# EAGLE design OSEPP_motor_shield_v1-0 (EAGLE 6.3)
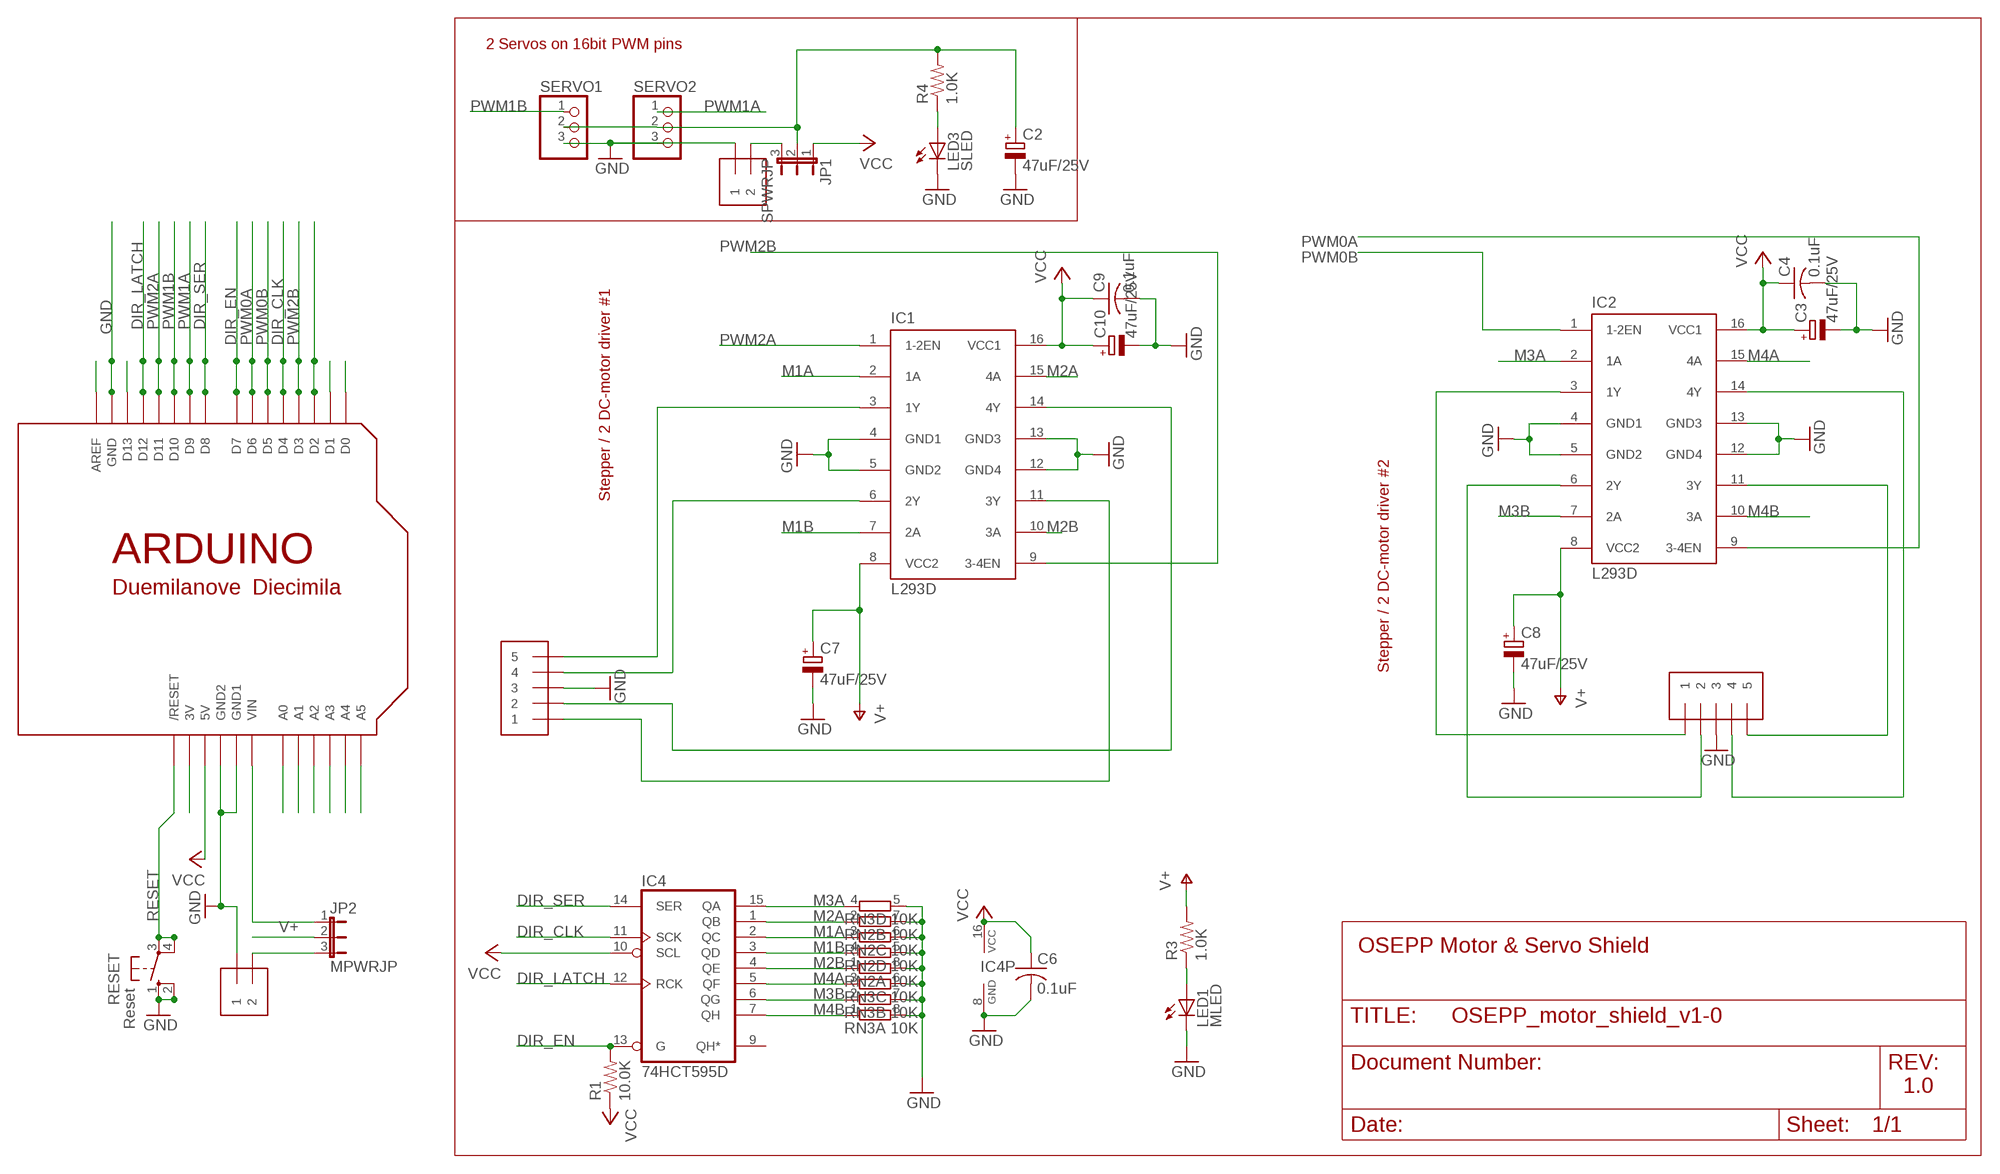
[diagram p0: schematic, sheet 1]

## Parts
C2  47uF/25V  CPOL-EUD  [PANASONIC_D]
C3  47uF/25V  CPOL-EUD  [PANASONIC_D]
C4  0.1uF  C-USC0603  [C0603]
C6  0.1uF  C-USC0603  [C0603]
C7  47uF/25V  CPOL-EUD  [PANASONIC_D]
C8  47uF/25V  CPOL-EUD  [PANASONIC_D]
C9  0.1uF  C-USC0603  [C0603]
C10  47uF/25V  CPOL-EUD  [PANASONIC_D]
IC1  L293D  L293E  [DIL16]
IC2  L293D  L293E  [DIL16]
IC4  74HCT595D  [SO16]
J1  1X5  [1X05-3.5MM]
J2  1X5  [1X05-3.5MM]
J3  1X2-3.5MM  [1X2-3.5MM]
J5  1X2-3.5MM  [1X2-3.5MM]
JP1  SPWRJP  JP2E  [JP2]
JP2  MPWRJP  JP2E  [JP2]
LED1  MLED  LEDCHIPLED_0805  [CHIPLED_0805]
LED3  SLED  LEDCHIPLED_0805  [CHIPLED_0805]
R1  10.0K  R-US_R0603  [R0603]
R3  1.0K  R-US_R0603  [R0603]
R4  1.0K  R-US_R0603  [R0603]
RESET  Reset  10-XX  [B3F-10XX]
RN2  10K  4R-NCAY16  [CAY16]
RN3  10K  4R-NCAY16  [CAY16]
SERVO1  PINHD-1X3  [1X03]
SERVO2  PINHD-1X3  [1X03]
U$1  ARDUINO-NOHOLE  [ARDUINO-NOHOLE]

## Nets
9V: JP2.1 U$1.VIN
DIR_CLK: IC4.11(SCK) U$1.D4
DIR_EN: IC4.13(G) R1.2 U$1.D7
DIR_LATCH: IC4.12(RCK) U$1.D12
DIR_SER: IC4.14(SER) U$1.D8
GND [power]: C2.- C3.- C4.2 C6.2 C7.- C8.- C9.2 C10.- IC1.4(GND1) IC1.5(GND2) IC1.12(GND4) IC1.13(GND3) IC2.4(GND1) IC2.5(GND2) IC2.12(GND4) IC2.13(GND3) IC4.8(GND) J1.3 J2.3 J3.1 J5.1 LED1.C LED3.C RESET.1(S) RESET.2(S1) RN2.5 RN2.6 RN2.7 RN2.8 RN3.5 RN3.6 RN3.7 RN3.8 SERVO1.3 SERVO2.3 U$1.GND U$1.GND1 U$1.GND2
M1A: IC1.2(1A) IC4.2(QC) RN2.3
M1B: IC1.7(2A) IC4.3(QD) RN2.4
M2A: IC1.15(4A) IC4.1(QB) RN2.2
M2B: IC1.10(3A) IC4.4(QE) RN2.1
M3A: IC2.2(1A) IC4.15(QA) RN3.4
M3B: IC2.7(2A) IC4.6(QG) RN3.2
M4A: IC2.15(4A) IC4.5(QF) RN3.3
M4B: IC2.10(3A) IC4.7(QH) RN3.1
N$1: IC1.3(1Y) J1.5
N$2: U$1.A0
N$3: U$1.A1
N$4: U$1.A2
N$5: U$1.A3
N$6: U$1.A4
N$7: IC2.3(1Y) J2.1
N$8: IC2.6(2Y) J2.2
N$9: IC2.11(3Y) J2.5
N$10: U$1.D2
N$11: U$1.D1
N$12: U$1.D0
N$13: U$1.A5
N$14: U$1.AREF
N$15: U$1.D13
N$16: LED1.A R3.1
N$17: U$1.3V
N$18: C2.+ JP1.2 R4.2 SERVO1.2 SERVO2.2
N$19: J3.2 JP2.3
N$20: IC2.14(4Y) J2.4
N$21: LED3.A R4.1
N$22: J5.2 JP1.3
N$31: IC1.6(2Y) J1.4
N$32: IC1.11(3Y) J1.1
N$33: IC1.14(4Y) J1.2
PWM0A: IC2.9(3-4EN) U$1.D6
PWM0B: IC2.1(1-2EN) U$1.D5
PWM1A: SERVO2.1 U$1.D9
PWM1B: SERVO1.1 U$1.D10
PWM2A: IC1.1(1-2EN) U$1.D11
PWM2B: IC1.9(3-4EN) U$1.D3
RESET: RESET.3(P) RESET.4(P1) U$1.RESET(/RESET)
V+: C7.+ C8.+ IC1.8(VCC2) IC2.8(VCC2) JP2.2 R3.2
VCC: C3.+ C4.1 C6.1 C9.1 C10.+ IC1.16(VCC1) IC2.16(VCC1) IC4.10(SCL) IC4.16(VCC) JP1.1 R1.1 U$1.5V
Unconnected: IC4.9(QH*)

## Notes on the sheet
- 2 Servos on 16bit PWM pins
- Stepper / 2 DC-motor driver #1
- Stepper / 2 DC-motor driver #2
- OSEPP Motor & Servo Shield
- 1.0

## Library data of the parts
C2 C3 C7 C8 C10 = rcl:CPOL-EU: POLARIZED CAPACITOR, European symbol
C4 C6 C9 = rcl:C-US: CAPACITOR, American symbol
IC1 IC2 = texas:L293E: TI DEVICE; MF: Arrow Electronics; MPN: L293E; OC_FARNELL: 1467711; OC_NEWARK: 89K0732
IC4 = 74xx-eu:74*595: 8-bit SHIFT REGISTER, output latch
J1 J2 = adafruit:1X5
J3 J5 = adafruit:1X2: 3.5mm Terminal block
JP1 JP2 = jumper:JP2E: JUMPER
LED1 LED3 = led:LED: LED
R1 R3 R4 = resistor:R-US_: RESISTOR, American symbol
RESET = switch-omron:10-XX: OMRON SWITCH; MPN: B3F-1000; OC_FARNELL: 176432; OC_NEWARK: 36M3542
RN2 RN3 = resistor-dil:4R-N: Array Chip Resistor Source: RS Component / Phycomp; OC_FARNELL: unknown; OC_NEWARK: unknown
SERVO1 SERVO2 = pinhead:PINHD-1X3: PIN HEADER
U$1 = adafruit:ARDUINO: Arduino Diecimila/Duemilanove Make a shield with ease, this package has all the named pins as well as the two mounting drill holes and an outline of the USB and DC power connector. The outline is on the DIMENSION layer, so if your board house uses it they will cut the outline to match.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

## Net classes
1 power: width 0.61 mm

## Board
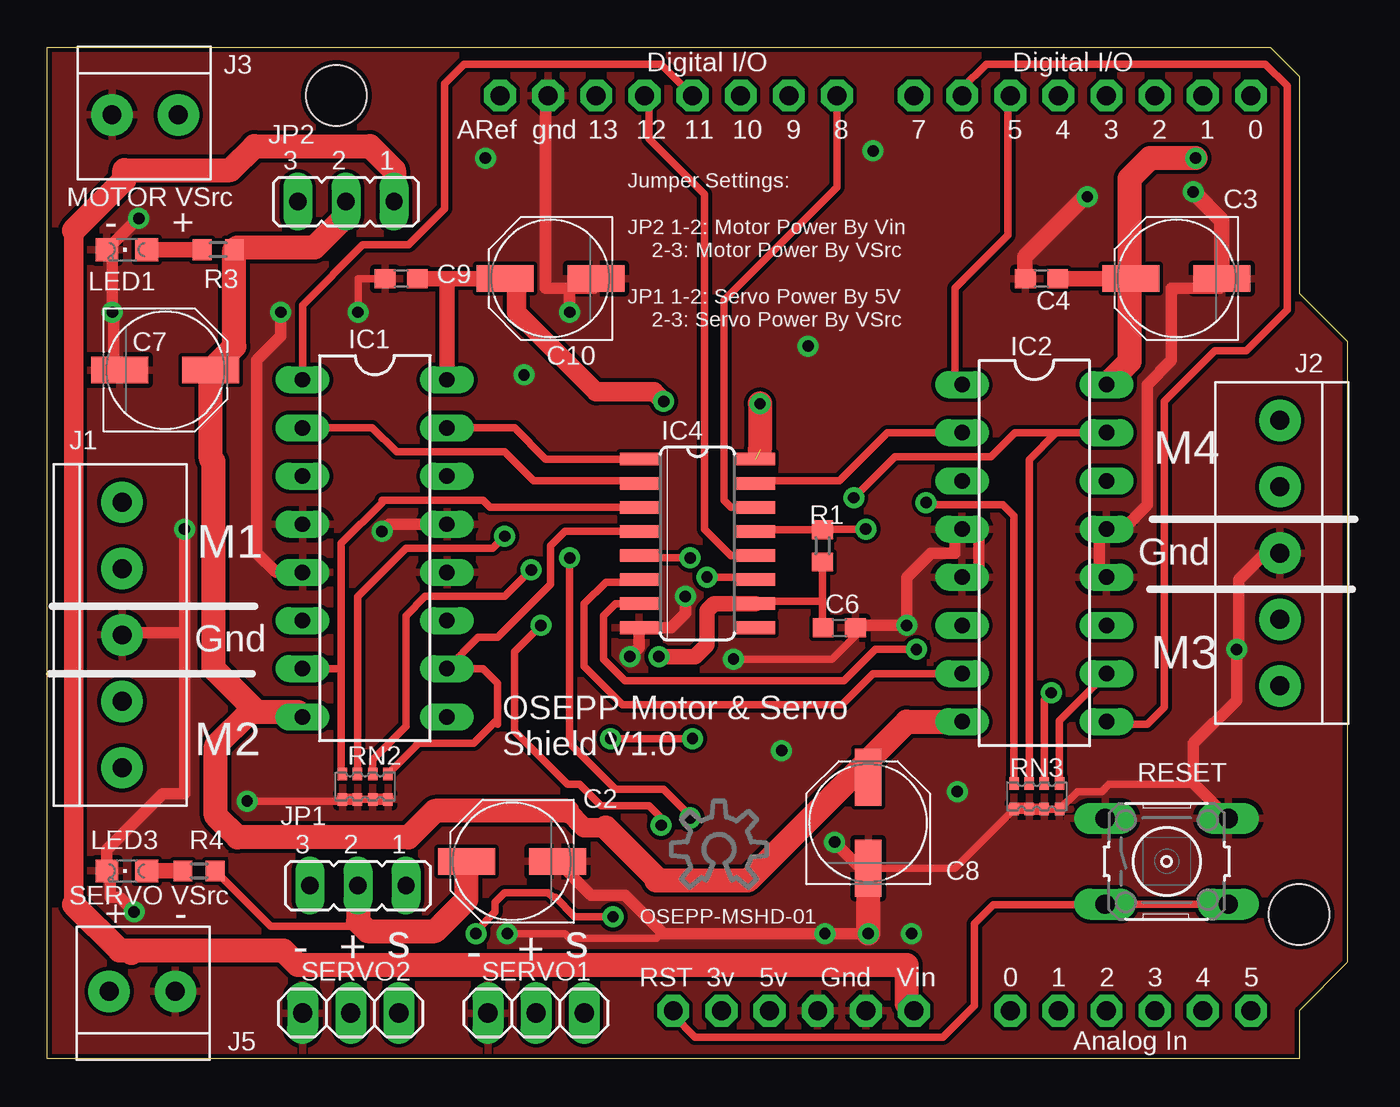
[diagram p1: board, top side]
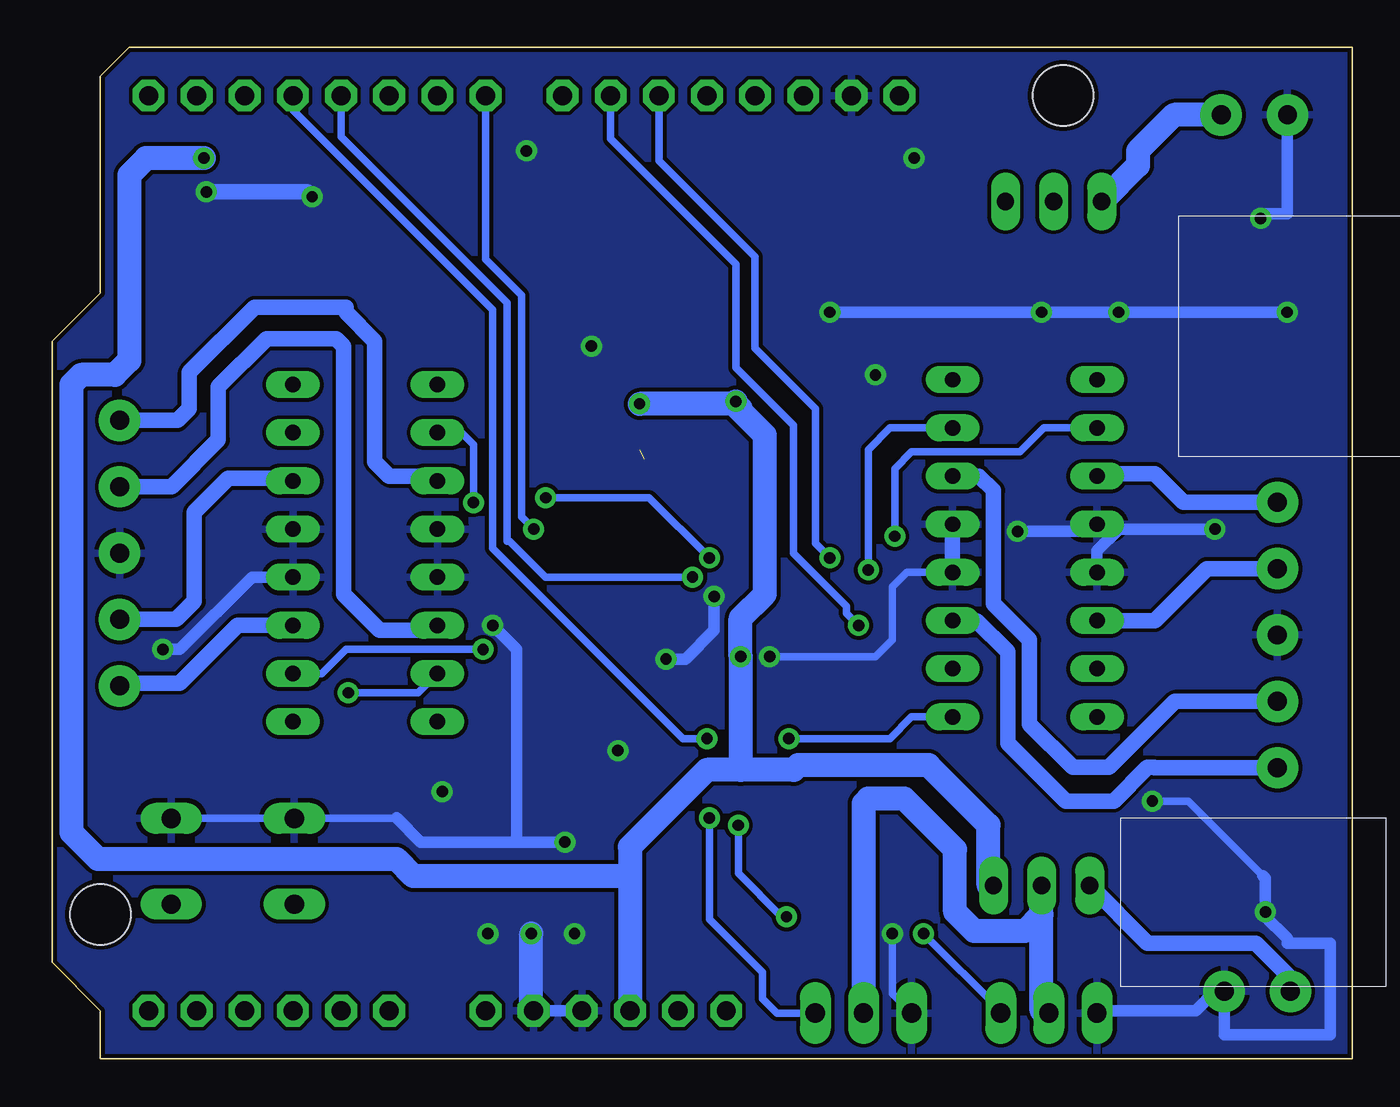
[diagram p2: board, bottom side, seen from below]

Size 68.58 x 53.34 mm. Coordinates in mm from the lower left corner, seen from the top.
Outline: 0,0 0,53.34 64.52,53.34 66.04,51.82 66.04,40.39 68.58,37.85 68.58,5.08 66.04,2.54 66.04,0 0,0
Copper layers (1*16): Top 0.035mm / dielectric 1.5mm / Bottom 0.035mm
Design rules "SparkFun": minimum track width 8mil, minimum drill 20mil, track to track 8mil, track to pad 8mil, pad to pad 8mil, via to via 8mil, smd to smd 8mil, copper to edge 10mil, drill to drill 8mil, minimum pad ring 12mil, minimum via ring 10mil, stop-mask expansion 4mil, vias tented up to drill 25mil, thermal gap 10mil
Holes 3.2 mm at 66.04,7.62 15.24,50.8

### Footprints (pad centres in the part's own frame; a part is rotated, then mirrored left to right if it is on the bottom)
PANASONIC_D = smd 3 x 1.4: + 2.4,0; - -2.4,0
C0603 = smd 1.1 x 1: 1 -0.85,0; 2 0.85,0
DIL16 = drill 0.813 long: 1 -8.89,-3.81; 2 -6.35,-3.81; 3 -3.81,-3.81; 4 -1.27,-3.81; 5 1.27,-3.81; 6 3.81,-3.81; 7 6.35,-3.81; 8 8.89,-3.81; 9 8.89,3.81; 10 6.35,3.81; 11 3.81,3.81; 12 1.27,3.81; 13 -1.27,3.81; 14 -3.81,3.81; 15 -6.35,3.81; 16 -8.89,3.81
SO16 = smd 0.66 x 2.032: 1 -4.445,-3.073; 2 -3.175,-3.073; 3 -1.905,-3.073; 4 -0.635,-3.073; 5 0.635,-3.073; 6 1.905,-3.073; 7 3.175,-3.073; 8 4.445,-3.073; 9 4.445,3.073; 10 3.175,3.073; 11 1.905,3.073; 12 0.635,3.073; 13 -0.635,3.073; 14 -1.905,3.073; 15 -3.175,3.073; 16 -4.445,3.073
1X05-3.5MM = drill 1 pad 2.184: 1 7,0; 2 3.5,0; 3 0,0; 4 -3.5,0; 5 -7,0
1X2-3.5MM = drill 1 pad 2.184: 1 1.8,0; 2 -1.7,0
JP2 = drill 0.914 long: 1 -2.54,0; 2 0,0; 3 2.54,0
CHIPLED_0805 = smd 1.2 x 1.2: A 0,-1.05; C 0,1.05
R0603 = smd 1 x 1.1: 1 -0.85,0; 2 0.85,0
B3F-10XX = drill 1.016 long: 1 -3.251,2.261; 2 3.251,2.261; 3 -3.251,-2.261; 4 3.251,-2.261
CAY16 = smd 0.5 x 0.65: 1 -1.2,-0.675; 2 -0.4,-0.675; 3 0.4,-0.675; 4 1.2,-0.675; 5 1.2,0.675; 6 0.4,0.675; 7 -0.4,0.675; 8 -1.2,0.675
1X03 = drill 1.016 long: 1 -2.54,0; 2 0,0; 3 2.54,0
ARDUINO-NOHOLE = drill 1 pad 1.676 octagon: 3V 35.56,2.54; 5V 38.1,2.54; A0 50.8,2.54; A1 53.34,2.54; A2 55.88,2.54; A3 58.42,2.54; A4 60.96,2.54; A5 63.5,2.54; AREF 23.876,50.8; D0 63.5,50.8; D1 60.96,50.8; D2 58.42,50.8; D3 55.88,50.8; D4 53.34,50.8; D5 50.8,50.8; D6 48.26,50.8; D7 45.72,50.8; D8 41.656,50.8; D9 39.116,50.8; D10 36.576,50.8; D11 34.036,50.8; D12 31.496,50.8; D13 28.956,50.8; GND 26.416,50.8; GND1 43.18,2.54; GND2 40.64,2.54; RESET 33.02,2.54; VIN 45.72,2.54

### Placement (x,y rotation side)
C2  24.51,10.41 180 top
C3  59.56,41.15 180 top
C4  52.45,41.15 180 top
C6  41.78,22.73 0 top
C7  6.22,36.32 0 top
C8  43.31,12.45 90 top
C9  18.67,41.15 180 top
C10  26.54,41.15 180 top
E$1  [OSHWLOGO_TOL_0.2]  35.43,11.05 0 top
IC1  17.27,26.92 270 top
IC2  52.07,26.67 270 top
IC4  34.29,27.18 270 top
J1  3.94,22.35 270 top
J2  65.02,26.67 90 top
J3  5.21,49.78 180 top
J5  4.95,3.56 0 top
JP1  16.38,9.14 180 top
JP2  15.75,45.21 180 top
LED1  4.19,42.67 90 top
LED3  4.19,9.91 90 top
R1  40.89,27.05 90 top
R3  9.02,42.67 0 top
R4  8,9.91 0 top
RESET  59.05,10.41 0 top
RN2  16.76,14.35 180 top
RN3  52.2,13.84 180 top
SERVO1  25.78,2.41 180 top
SERVO2  16,2.41 180 top
U$1  0,0 0 top

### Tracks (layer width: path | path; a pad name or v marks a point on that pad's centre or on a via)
9V
  Top 1.016: 1.4,8.13 1.4,43.69
  Top 1.27: U$1.VIN 45.34,2.92 45.34,4.95 13.21,4.95 12.45,5.71 4.57,5.71 | 1.4,43.69 4.06,46.35 4.06,46.86 9.65,46.86 10.92,48.13 17.02,48.13 18.29,46.86 JP2.1 | 4.44,5.59 4.57,5.71 | 1.4,8.13 3.81,5.71 4.57,5.71
DIR_CLK  (via drill 0.6)
  Top 0.406: v34.8,25.4 37.24,25.4 IC4.11
  Bottom 0.406: v34.8,25.4 42.55,25.4 44.45,27.3 44.58,27.3 44.58,39.88 53.34,48.64 U$1.D4
DIR_EN  (via drill 0.6)
  Top 0.406: IC4.13 37.45,27.9 R1.2 40.93,27.94 v43.18,27.94
  Bottom 0.406: U$1.D7 45.72,42.16 43.81,40.26 43.81,28.57 v43.18,27.94
DIR_LATCH
  Top 0.406: IC4.12 36.07,26.54 34.67,27.94 34.67,45.59 31.75,48.51 31.75,50.55 U$1.D12
DIR_SER
  Top 0.406: IC4.14 36.07,29.08 35.69,29.46 35.69,40.01 41.66,45.97 U$1.D8
GND  (via drill 0.6)
  Top 0.406: C9.2 16.38,41.15 v16.38,39.37 | RN3.7 RN3.8 54.33,14.1 55.63,14.1 56.01,14.48 60.58,14.48 | RN3.6 RN3.5 47.88,10.05 C8.- | RN2.7 RN2.6 | RN2.5 15.48,13.59 v10.54,13.59 | 32.38,6.6 32.13,6.35 27.56,6.35 27.3,6.6 v24.26,6.6 | v36.2,21.08 41.4,21.08 42.63,22.31 C6.2
  Top 0.61: 27.56,40.64 26.29,40.64 26.29,50.8 U$1.GND | 27.56,40.64 28.83,40.64 | 3.43,36.83 3.5,36.73 | 3.5,36.73 C7.- | IC2.12 55.5,25.4 55.5,27.94 IC2.13 56.77,27.94 58.04,29.21 58.04,35.56 59.31,36.83 59.31,40.64 61.85,40.64 C3.- | C6.2 42.8,22.86 v45.34,22.86 45.34,25.4 46.61,26.67 47.88,26.67 47.88,27.94 IC2.4 49.15,27.94 49.15,25.4 IC2.5 | C8.- 42.8,10.16 v41.53,11.43 | C2.- 28.69,8.64 30.48,8.64 32.38,6.73 32.38,6.6 v41.02,6.6 v43.31,6.6 | RN2.6 RN2.5 | RN2.7 RN2.8 | RN3.7 RN3.6 51.76,13.21 50.93,13.21 | IC1.5 12.06,25.65 11.05,26.67 11.05,36.83 12.32,38.1 v12.32,39.37 | v17.65,27.81 18.03,28.19 IC1.13 | J2.3 64.26,26.67 62.87,25.27 62.87,21.72 v62.74,21.59 62.74,18.92 60.45,16.64 60.45,14.53 RESET.2 | 3.5,36.73 3.5,39.3 v3.43,39.37 3.43,42.16 3.14,42.45 LED1.C 4.79,44.32 v4.83,44.32 | v7.24,27.94 7.24,22.48 | 7.24,22.48 7.24,13.97 6.1,13.97 3.14,11.02 LED3.C 3.3,9.74 3.3,8.51 3.81,8.51 v4.57,7.75 | J1.3 4.06,22.48 7.24,22.48 | v30.73,21.21 31.22,21.69 IC4.8 32.89,22.73 33.66,23.5 v33.66,24.38 | C10.- 29.72,41.15 | v27.56,39.37 27.56,40.64
  Top 0.813: C4.2 51.56,41.19 51.56,42.29 54.74,45.47 v54.86,45.47 | v60.45,45.72 61.96,44.21 C3.-
  Top 1.27: v43.31,6.6 C8.-
  Bottom 0.406: IC1.12 23.5,25.65 24.26,24.89 24.26,22.1 25.15,21.21 v30.73,21.21 | v10.54,13.59 8.64,13.59 4.7,9.65 | 50.42,12.7 50.44,12.68 RESET.1 RESET.2 | 61.85,12.7 61.98,12.7 | SERVO1.3 24.26,3.43 v24.26,6.6
  Bottom 0.61: SERVO2.3 13.59,2.54 8.25,2.54 7.24,3.56 J5.1 6.73,3.56 6.73,1.27 1.14,1.27 1.14,6.1 3.43,6.1 3.43,6.35 4.57,7.49 v4.57,7.75 4.57,9.53 4.7,9.65 | v7.24,27.94 12.32,27.94 | U$1.GND1 U$1.GND2 40.26,2.54 | 44.07,11.43 49.15,11.43 50.42,12.7 | 44.07,11.43 44.07,21.59 v45.34,22.86 | IC2.12 58.04,25.4 61.85,21.59 v62.74,21.59 | v36.2,21.08 35.18,21.08 33.66,22.61 v33.66,24.38 | 12.32,27.94 12.57,28.19 IC1.4 13.84,27.81 v17.65,27.81 | 12.32,27.94 13.46,26.8 IC1.5 | v3.43,39.37 v12.32,39.37 v16.38,39.37 v27.56,39.37 | v41.53,11.43 44.07,11.43 | v4.83,44.32 4.57,44.58 3.43,44.58 3.41,44.6 J3.1
  Bottom 0.813: v54.86,45.47 55.12,45.72 v60.45,45.72 | IC1.13 IC1.12
  Bottom 1.27: U$1.GND1 43.31,2.67 v43.31,6.6
  other vias: 23.11,47.5 43.56,47.88 48.01,14.1 38.73,16.26 40.13,37.59 25.15,36.07 45.59,6.6
  pour Bottom: -0.64,53.85 -0.64,-1.02 69.22,-1.02 69.22,53.98 -0.64,53.98
  pour Top: -0.64,53.98 -0.76,53.85 -0.64,-1.02 69.22,-1.02 69.22,53.98
M1A  (via drill 0.6)
  Top 0.254: 31.09,30.48 IC4.2
  Top 0.406: IC1.2 17.14,33.27 18.41,32 24.13,32 25.65,30.48 31.09,30.48 | RN2.3 16.36,24.36 18.92,26.92 23.5,26.92 v24.13,27.56
  Bottom 0.406: v24.13,27.56 24.13,31.11 23.24,32 17.53,32 16.26,33.27 IC1.2
M1B
  Top 0.406: IC1.7 15.49,20.57 | 15.49,20.57 15.49,27.18 17.65,29.34 17.65,29.46 22.99,29.46 23.37,29.08 IC4.3 | RN2.4 15.49,15.1 15.49,20.57
M2A  (via drill 0.6)
  Top 0.406: IC1.15 24.64,33.27 26.29,31.62 IC4.1 | RN2.2 17.16,15.77 18.92,17.53 18.92,23.37 19.94,24.38 24.13,24.38 v25.53,25.78
  Bottom 0.406: v25.53,25.78 25.53,32.13 24.38,33.27 IC1.15
M2B
  Top 0.406: IC4.4 27.3,27.81 26.54,27.05 26.54,25.02 23.75,22.23 22.73,22.23 IC1.10 22.99,20.57 23.75,19.81 23.75,18.16 23.75,17.91 | 23.75,17.65 23.75,17.91 | RN2.1 19.47,16.53 19.47,16.55 19.56,16.64 22.48,16.64 23.75,17.91
M3A  (via drill 0.6)
  Top 0.254: 37.49,30.48 IC4.15
  Top 0.406: IC2.2 44.32,33.02 41.78,30.48 37.49,30.48 | RN3.4 51,28.63 50.42,29.21 46.48,29.21 v46.35,29.34
  Bottom 0.406: 47.24,33.02 IC2.2 46.99,33.02 46.35,32.38 v46.35,29.34
M3B  (via drill 0.6)
  Top 0.254: IC2.7 48.39,20.32
  Top 0.406: IC2.7 43.56,20.32 41.91,18.67 30.35,18.67 28.32,20.7 28.32,24 29.46,25.15 31.09,25.15 IC4.6 | RN3.2 52.6,18.94 v52.96,19.3
  Bottom 0.406: v52.96,19.3 49.28,19.3 IC2.7
M4A  (via drill 0.6)
  Top 0.406: IC2.15 53.21,33.02 | 53.21,33.02 51.05,33.02 49.78,31.75 44.7,31.75 v42.55,29.59 | v33.91,26.42 31.34,26.42 IC4.5 | RN3.3 51.8,31.6 53.21,33.02
  Bottom 0.406: v42.55,29.59 37.08,29.59 v33.91,26.42
M4B  (via drill 0.6)
  Top 0.406: RN3.1 53.4,17.84 IC2.10 | IC4.7 29.97,24 29.34,23.37 29.34,21.08 30.48,19.94 42.04,19.94 43.69,21.59 v45.85,21.59
  Bottom 0.406: v45.85,21.59 53.09,21.59 54.36,20.32 IC2.10 55.63,20.07
N$1
  Bottom 0.813: J1.5 8.9,29.35 10.41,30.86 13.33,30.86 IC1.3
N$7
  Bottom 0.813: J2.1 61.96,33.67 61.34,34.29 61.34,36.2 57.91,39.62 53.09,39.62 53.09,39.37 51.56,37.85 51.56,31.5 50.8,30.73 48.51,30.73 IC2.3
N$8
  Bottom 0.813: J2.2 62.29,30.17 59.82,32.64 59.82,35.43 57.28,37.97 53.59,37.97 53.21,37.59 53.21,24.51 51.31,22.61 48.51,22.61 IC2.6
N$9
  Bottom 0.813: IC2.11 58.8,22.86 61.85,19.81 64.88,19.81 J2.5
N$16
  Top 0.813: LED1.A R3.1
N$18
  Top 0.406: R4.2 11.77,6.99 16.38,6.99 JP1.2
  Top 1.27: JP1.2 16.38,7.24 16.89,6.73 20.45,6.73 22.11,8.39 C2.+
  Bottom 1.27: SERVO2.2 16.13,2.29 16.38,2.54 JP1.2 16.38,7.62 17.27,6.73 19.94,6.73 20.95,7.75 20.95,11.05 23.62,13.72 25.53,13.72 25.78,13.46 SERVO1.2
N$19
  Bottom 1.27: J3.2 9.4,49.78 11.3,47.88 11.3,47.12 JP2.3
N$20
  Bottom 0.813: J2.4 62.05,23.17 61.09,24.13 61.09,28.83 59.31,30.61 56.01,30.61 IC2.14
N$21
  Top 0.813: R4.1 LED3.A
N$22
  Bottom 0.813: J5.2 3.25,4.27 5.08,6.1 10.79,6.1 JP1.3
N$31
  Bottom 0.813: J1.4 7.68,25.85 10.41,23.11 IC1.6
N$32
  Bottom 0.813: J1.1 10.43,15.35 10.44,15.37 10.79,15.37 12.57,13.59 15.11,13.59 18.16,16.64 18.16,21.46 19.81,23.11 IC1.11
N$33
  Bottom 0.813: J1.2 9.34,18.85 12.83,15.37 14.73,15.37 17.02,17.65 17.02,22.1 18.92,24 18.92,29.97 19.68,30.73 IC1.14 20.83,30.48
PWM0A
  Top 0.406: U$1.D6 48.26,51.18 49.53,52.45 64.26,52.45 65.41,51.31 65.41,39.5 63.25,37.34 61.59,37.34 58.93,34.67 58.93,18.54 58.04,17.65 56.01,17.65 IC2.9
PWM0B
  Top 0.406: U$1.D5 50.67,50.93 50.67,43.43 47.88,40.64 47.88,35.94 IC2.1
PWM1A  (via drill 0.6)
  Top 0.406: v22.61,6.6 22.61,6.73 23.62,7.75 23.62,8.26 24.13,8.76 26.42,8.76 26.67,8.51 26.8,8.51 27.81,7.49 v29.84,7.49 | v32.38,12.32 32.38,12.7 31.75,13.34 29.21,13.34 28.07,14.48 27.43,14.48 24.64,17.27 24.64,21.46 v26.04,22.86
  Bottom 0.406: U$1.D9 39.12,48.51 32.51,41.91 32.51,36.45 29.46,33.4 29.46,26.67 26.67,23.88 26.67,23.5 v26.04,22.86 | v22.61,6.6 18.54,2.54 SERVO2.1 | 29.97,7.62 v29.84,7.49 30.1,7.49 32.38,9.78 v32.38,12.32
PWM1B  (via drill 0.6)
  Top 0.406: v27.56,26.42 27.56,16.64 29.97,14.22 32.51,14.22 33.91,12.83 v33.91,12.7
  Bottom 0.406: SERVO1.1 30.35,2.41 31.11,3.17 31.11,4.57 33.91,7.37 v33.91,12.7 | v27.56,26.42 28.32,27.18 28.32,34.29 31.5,37.47 31.5,42.29 36.58,47.37 U$1.D10
PWM2A
  Top 0.406: IC1.1 13.46,39.75 16.64,42.93 19.05,42.93 20.95,44.83 20.95,51.44 21.97,52.45 32.38,52.45 U$1.D11
PWM2B  (via drill 0.6)
  Top 0.406: v29.72,16.89 v34.04,16.89
  Bottom 0.406: v29.72,16.89 24.38,16.89 23.24,18.03 IC1.9 | v34.04,16.89 35.31,16.89 45.34,26.92 45.34,39.5 55.88,50.04 U$1.D3
RESET
  Top 0.406: U$1.RESET 33.02,2.29 34.16,1.14 47.24,1.14 48.9,2.79 48.9,7.11 49.91,8.13 55.78,8.13 RESET.3 RESET.4
V+
  Top 0.813: 9.91,40.26 9.91,42.63 | 9.91,42.63 R3.2 | 9.91,42.63 9.91,42.67 10.03,42.8 | 15.75,44.45 JP2.2 | C8.+ 43.31,15.75 | 48.01,17.53 IC2.8
  Top 1.016: 27.43,13.08 28.32,12.19 29.46,12.19 | 32.13,9.53 32.13,9.4
  Top 1.27: 10.03,42.8 14.1,42.8 15.75,44.45 | 32.13,9.4 36.96,9.4 43.31,15.75 45.34,17.78 IC2.8 | 27.43,13.08 20.45,13.08 19.05,11.68 10.03,11.68 8.89,12.83 8.89,16.51 10.67,18.29 10.67,18.67 | IC1.8 13.21,18.29 11.05,18.29 10.67,18.67 | 10.67,18.67 8.76,20.57 8.76,31.5 8.62,31.64 C7.+ 9.87,37.57 R3.2 | 29.46,12.19 32.13,9.53
VCC  (via drill 0.6)  (1 unrouted)
  Top 0.406: R1.1 40.89,24 | 40.89,24 40.89,22.77 C6.1 | IC4.10 37.97,24 38.1,24.13 40.77,24.13 40.89,24
  Top 0.813: 21.21,41.15 C10.+ 24.38,41.15 24.77,40.77 | 21.21,41.15 C9.1 | IC1.16 21.08,41.02 21.21,41.15 | IC2.16 57.09,36.77 57.16,36.84 C3.+ C4.1 | IC4.10 35.18,24 34.8,23.62 34.8,21.84 34.16,21.21 v32.26,21.21 | v37.59,34.54 37.62,34.57
  Top 1.016: v32.51,34.67 32,35.18 28.96,35.18 24.77,39.37 24.77,40.77
  Top 1.27: IC2.16 56.9,36.58 | v60.58,47.5 58.17,47.5 57.09,46.42 57.09,36.77 | 37.62,34.57 37.59,34.57 37.59,32.13
  Bottom 0.813: U$1.5V 38.1,5.08 | v32.51,34.67 32.64,34.54
  Bottom 1.27: v60.58,47.5 63.63,47.5 64.52,46.61 64.52,36.83 65.28,36.07 67.06,36.07 67.56,35.56 67.56,11.94 66.17,10.54 50.42,10.54 49.53,9.65 38.1,9.65 | 32.26,15.24 v32.26,21.21 32.26,23.24 30.99,24.51 30.99,32.89 32.51,34.42 v32.51,34.67 32.51,34.54 32.26,34.29 | 38.1,9.65 U$1.5V | 32.26,15.24 29.46,15.24 29.21,15.49 22.35,15.49 19.18,12.32 19.18,9.14 JP1.1 | 32.26,15.24 34.04,15.24 38.1,11.18 38.1,9.65 | 32.64,34.54 v37.59,34.54

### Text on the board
tPlace: J3 | MOTOR VSrc | - | + | Jumper Settings: / / JP2 1-2: Motor Power By Vin / 2-3: Motor Power By VSrc / / JP1 1-2: Servo Power By 5V / 2-3: Servo Power By VSrc | M4 | M1 | Gnd | M3 | Gnd | M2 | OSEPP Motor & Servo / Shield V1.0 | SERVO VSrc | + | - | OSEPP-MSHD-01 | - | + | s | - | + | s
